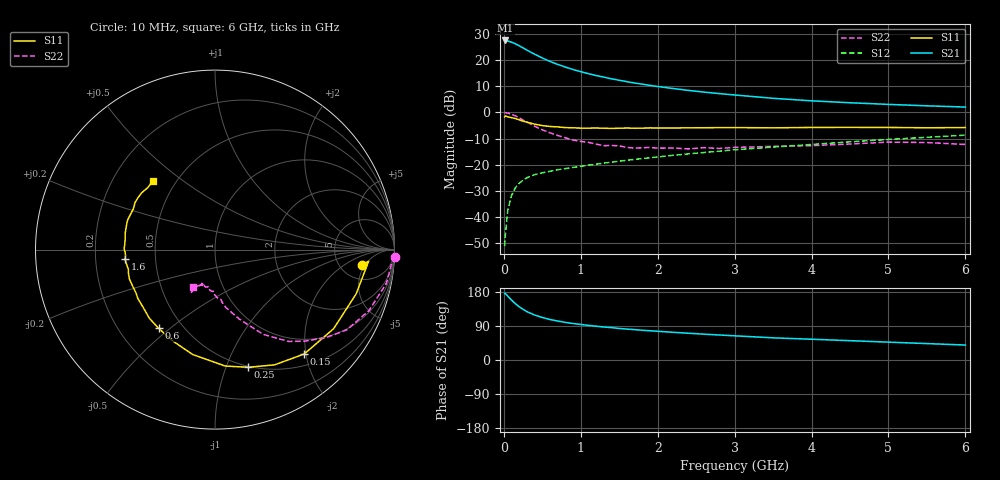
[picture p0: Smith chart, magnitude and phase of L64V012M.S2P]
!  INFINEON TECHNOLOGIES Small Signal Semiconductors
! BFR380L3 , Si-NPN RF-Transistor in TSLP-3-1
!  Vce=4 V,  Ic=12.5 mA
! Common Emitter S-Parameters:  07. March 2005
#  GHz  S  MA  R  50
! f  S11  S21  S12  S22
! GHz  Mag  Ang  Mag  Ang  Mag  Ang  Mag  Ang
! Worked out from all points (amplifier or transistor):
!   36 points, 10 MHz to 6 GHz, reference 50 ohm
!   highest |S21| = 27.5 dB at 20 MHz (marker M1)
!   |S21| within 3 dB of that: start of sweep to 259.1 MHz
!   unconditionally stable (mu >= 1): 2.277 GHz to 4.71 GHz
!   at 250 MHz: K = 0.26, MSG = 25.3 dB, |S12| = -25.9 dB
!   at 1.4 GHz: K = 0.88, MSG = 15.9 dB, |S12| = -19.0 dB
!   at 6 GHz: K = 0.96, MSG = 5.4 dB, |S12| = -8.7 dB
!   S11 on the Smith chart (normalised r, x): 10 MHz: 8.08, -4.26; 150 MHz: 0.70, -1.97; 250 MHz: 0.49, -1.20; 600 MHz: 0.37, -0.46; 1.6 GHz: 0.33, -0.05; 6 GHz: 0.38, +0.39
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0.01  0.8239 -5.9  23.63 175.8  0.0028 87.3  1.005 -2.3
0.02  0.8584 -4.3  23.66 175.5  0.0046 85.0  0.9867 -4.6
0.05  0.8243 -17.4  23.13 168.6  0.0132 83.7  0.9729 -11.2
0.1  0.7944 -33.7  21.91 158.1  0.026 74.4  0.9224 -21.7
0.15  0.7651 -49.5  20.45 148.5  0.0365 66.9  0.8598 -31.3
0.2  0.7227 -62.7  18.7 140.4  0.0445 61.9  0.7887 -38.5
0.25  0.6811 -74.3  17.05 133.7  0.0508 57.8  0.7138 -45.6
0.3  0.6512 -85.0  15.46 127.7  0.0567 55.2  0.6557 -51.3
0.4  0.5976 -102.0  12.92 118.7  0.0648 51.1  0.5442 -60.3
0.5  0.5605 -115.0  10.96 112.2  0.0705 49.4  0.4654 -65.6
0.6  0.5394 -125.6  9.402 106.9  0.0752 48.5  0.4091 -70.8
0.7  0.5294 -133.7  8.261 102.8  0.0805 49.5  0.3632 -75.1
0.8  0.5135 -141.3  7.348 99.2  0.0848 49.2  0.3282 -79.4
0.9  0.5088 -147.8  6.59 96.3  0.0891 50.2  0.2965 -82.3
1.1  0.5021 -156.5  5.495 91.3  0.0987 51.4  0.2685 -87.4
1.4  0.4949 -167.3  4.386 85.4  0.1122 53.9  0.2338 -93.3
1.6  0.5046 -174.0  3.866 81.6  0.122 54.9  0.2145 -100.4
2.2  0.504 173.5  2.863 73.1  0.1519 58.1  0.2091 -105.8
3.5  0.5084 153.6  1.861 58.5  0.218 59.9  0.2251 -115.7
4.5  0.5174 146.2  1.531 51.0  0.2748 60.5  0.2496 -117.9
5.5  0.5096 137.5  1.337 43.3  0.3358 58.5  0.2663 -119.4
6  0.5146 132.1  1.267 39.5  0.3686 56.9  0.2448 -120.7
